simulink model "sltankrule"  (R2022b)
settings: Solver=ode45  StartTime=0  StopTime=Inf  MaxStep=0.2  RelTol=1e-3  AbsTol=1e-6
PreLoadFcn:
  | tank = readfis('tank');
libraries: fuzblock x1, slpidlib x1

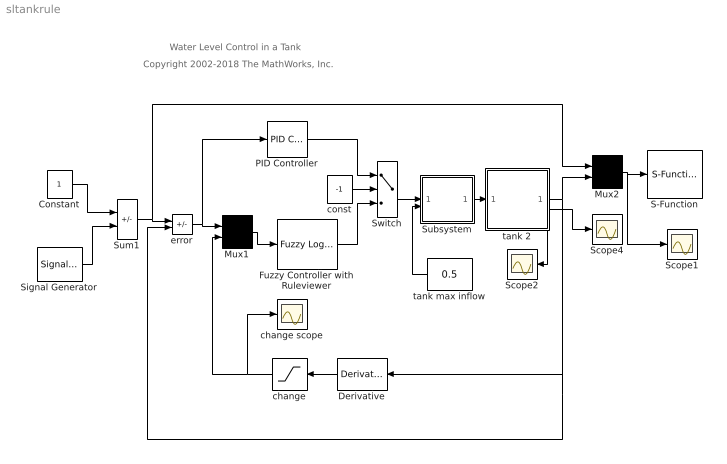
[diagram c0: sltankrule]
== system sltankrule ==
  note: Water Level Control in a Tank
  note: Copyright 2002-2018 The MathWorks, Inc.
  Constant : Constant
  Derivative : Derivative
  Fuzzy Controller with Ruleviewer : fuzblock/Fuzzy Logic  Controller  with Ruleviewer  fismatrix=tank  Ts=2
  Mux1 : Mux  Inputs=2
  Mux2 : Mux  Inputs=2
  PID Controller : slpidlib/PID Controller  Controller=PID  Form=Parallel  TimeDomain=Continuous-time  UseExternalTs=off  SampleTime=1  IntegratorMethod=Forward Euler  FilterMethod=Forward Euler  ControllerParametersSource=internal  P=2  I=0  UseKiTs=off  D=1  N=100  UseFilter=on  TunerSelectOption=Transfer Function Based (PID Tuner App)  InitialConditionSource=internal  InitialConditionForIntegrator=0  InitialConditionForFilter=0  DifferentiatorICPrevScaledInput=0  ExternalReset=none  TrackingMode=off  Kt=1  LimitOutput=off  SatLimitsSource=internal  UpperSaturationLimit=inf  LowerSaturationLimit=-inf  LinearizeAsGain=off  AntiWindupMode=none  Kb=1  LimitIntegrator=off  UpperIntegratorSaturationLimit=inf  LowerIntegratorSaturationLimit=-inf  POutMin=[]  POutMax=[]  IOutMin=[]  IOutMax=[]  DOutMin=[]  DOutMax=[]  NOutMin=[]  NOutMax=[]  SumOutMin=[]  SumOutMax=[]  SaturationOutMin=[]  SaturationOutMax=[]  PParamMin=[]  PParamMax=[]  IParamMin=[]  IParamMax=[]  DParamMin=[]  DParamMax=[]  NParamMin=[]  NParamMax=[]  KbParamMin=[]  KbParamMax=[]  KtParamMin=[]  KtParamMax=[]  KbOutMin=[]  KbOutMax=[]  KtOutMin=[]  KtOutMax=[]  IntegratorOutMin=[]  IntegratorOutMax=[]  FilterOutMin=[]  FilterOutMax=[]  SumI1OutMin=[]  SumI1OutMax=[]  SumI2OutMin=[]  SumI2OutMax=[]  SumI3OutMin=[]  SumI3OutMax=[]  SumI4OutMin=[]  SumI4OutMax=[]  SumDOutMin=[]  SumDOutMax=[]  DifferentiatorOutMin=[]  DifferentiatorOutMax=[]  FilterDiffOutCoefMin=[]  FilterDiffOutCoefMax=[]  ReciprocalOutMin=[]  ReciprocalOutMax=[]  SumDenOutMin=[]  SumDenOutMax=[]  SumNumOutMin=[]  SumNumOutMax=[]  DivideOutMin=[]  DivideOutMax=[]  UdiffTsProdOutMin=[]  UdiffTsProdOutMax=[]  NTsProdOutMin=[]  NTsProdOutMax=[]  UintegralTsProdOutMin=[]  UintegralTsProdOutMax=[]  UngainTsProdOutMin=[]  UngainTsProdOutMax=[]  ClampingZeroOutDataTypeStr=Inherit: Inherit via back propagation  ClampingZeroOutMin=[]  ClampingZeroOutMax=[]  FilterDenConstantOutDataTypeStr=Inherit: Inherit via back propagation  FilterDenConstantOutMin=[]  FilterDenConstantOutMax=[]  PCopyOutDataTypeStr=Inherit: Inherit via back propagation  PCopyOutMin=[]  PCopyOutMax=[]  NCopyOutDataTypeStr=Inherit: Inherit via back propagation  NCopyOutMin=[]  NCopyOutMax=[]  IntegratorContinuousStateAttributes=''  IntegratorStateMustResolveToSignalObject=off  IntegratorRTWStateStorageClass=Auto  FilterContinuousStateAttributes=''  FilterStateMustResolveToSignalObject=off  FilterRTWStateStorageClass=Auto  ParallelPVariant=InternalParameters  IdealPVariant=Disabled  IVariant=InternalParameters  DVariant=InternalParameters  IntegratorVariant=Continuous  SatVariant=Disabled  AWVariant=Passthrough  PCopyVariant=Disabled  TRVariant=Disabled  FdbkBlocksVariant=Forward  IdealPFdbkVariant=Disabled  SatFdbkVariant=Disabled  DerivativeFilterVariant=ContFilter  NVariant=InternalParameters  NCopyVariant=Disabled  FilterICVariant=InternalICsFilter  IntegratorICVariant=InternalICs  ExternalResetVariant=Disabled  TRSumVariant=Passthrough  SumFdbkVariant=Disabled  SumVariant=Sum_PID  TsampFilterVariant=InternalTs  TsampNgainVariant=Passthrough  TsampIntegralVariant=Passthrough  ExternalSaturationOutDataTypeStr=Inherit: Same as second input
  S-Function : S-Function  FunctionName=animtank  Parameters=1  SFunctionDeploymentMode=off  EnableBusSupport=off
  Scope1 : Scope
  Scope2 : Scope
  Scope4 : Scope
  Signal Generator : SignalGenerator  WaveForm=square  Amplitude=0.500000  Frequency=0.100000  Units=rad/sec
  Subsystem : Subsystem  mask(Valve){InitialPosition=0}
      mask prompts: InitialPosition "Initial position [0=closed 1=open]:"
      mask help: Valve
  Sum1 : Sum  Inputs=+-  InputSameDT=on  SaturateOnIntegerOverflow=on
  Switch : Switch
  change : Saturate  UpperLimit=0.1  LowerLimit=-0.1
  change scope : Scope
  const : Constant  Value=-1
  error : Sum  Inputs=+-  InputSameDT=on  SaturateOnIntegerOverflow=on
  tank 2 : Subsystem  mask(Water tank){ht=2, area=1, outletArea=0.05, overflowLimit=0, initialHt=0.5}
      mask prompts: ht "Height of tank (m):"; area "Bottom area (m^2):"; outletArea "Out pipe crossection (m^2):"; overflowLimit "Overflow sensor distance from top (m):"; initialHt "Initial level height (m):"
      mask help: Cylindrical water tank with overflow signal
  tank max inflow : Constant  Value=0.5
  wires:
  tank 2/2(flow out) -> Scope4/1
  tank max inflow/1 -> Subsystem/2(source flow)
  Derivative/1 -> change/1
  Mux1/1 -> Fuzzy Controller with Ruleviewer/1
  change/1 -> Mux1/2, change scope/1
  Constant/1 -> Sum1/1
  Signal Generator/1 -> Sum1/2
  Subsystem/1(out flow) -> tank 2/1(flow in)
  tank 2/1(water level) -> Mux2/2, error/2, Derivative/1
  Sum1/1 -> error/1, Mux2/1
  tank 2/3(overflow flag) -> Scope2/1
  Switch/1 -> Subsystem/1(control)
  Mux2/1 -> S-Function/1, Scope1/1
  error/1 -> Mux1/1, PID Controller/1
  Fuzzy Controller with Ruleviewer/1 -> Switch/3
  PID Controller/1 -> Switch/1
  const/1 -> Switch/2

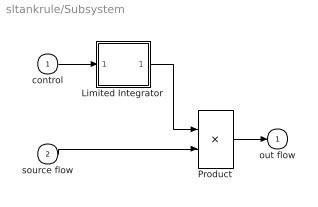
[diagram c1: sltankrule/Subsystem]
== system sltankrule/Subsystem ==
  control : Inport
  source flow : Inport  Port=2
  Limited Integrator : Subsystem  mask(Limited integrator.){lb=0, ub=1, xi=InitialPosition}
      mask prompts: lb "Lower bound:"; ub "Upper bound:"; xi "Initial condition"
      mask help: Limited integrator
  Product : Product  InputSameDT=on  RndMeth=Zero  SaturateOnIntegerOverflow=on
  out flow : Outport  InitialOutput=0  VectorParamsAs1DForOutWhenUnconnected=off
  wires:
  source flow/1 -> Product/2
  Product/1 -> out flow/1
  control/1 -> Limited Integrator/1(In_1)
  Limited Integrator/1(Out_1) -> Product/1

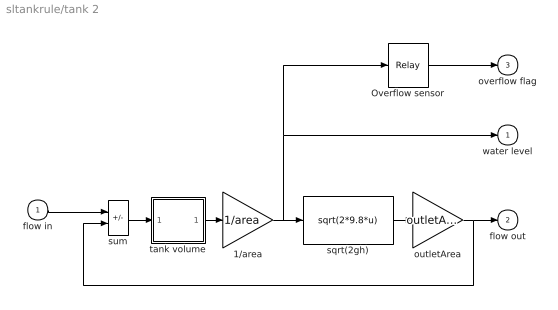
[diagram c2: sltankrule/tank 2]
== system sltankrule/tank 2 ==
  flow in : Inport
  1/area : Gain  Gain=1/area  SaturateOnIntegerOverflow=on
  Overflow sensor : Relay  OnSwitchValue=ht - overflowLimit  OffSwitchValue=ht - overflowLimit
  outletArea : Gain  Gain=outletArea  SaturateOnIntegerOverflow=on
  sqrt(2gh) : Fcn  Expr=sqrt(2*9.8*u)
  sum : Sum  Inputs=+-  InputSameDT=on  SaturateOnIntegerOverflow=on
  tank volume : Subsystem  mask(Limited integrator.){lb=0, ub=ht * area, xi=initialHt * area}
      mask prompts: lb "Lower bound:"; ub "Upper bound:"; xi "Initial condition"
      mask help: Limited integrator
  water level : Outport  InitialOutput=0  VectorParamsAs1DForOutWhenUnconnected=off
  flow out : Outport  Port=2  InitialOutput=0  VectorParamsAs1DForOutWhenUnconnected=off
  overflow flag : Outport  Port=3  InitialOutput=0  VectorParamsAs1DForOutWhenUnconnected=off
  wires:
  outletArea/1 -> flow out/1, sum/2
  sqrt(2gh)/1 -> outletArea/1
  1/area/1 -> Overflow sensor/1, water level/1, sqrt(2gh)/1
  tank volume/1(Out_1) -> 1/area/1
  Overflow sensor/1 -> overflow flag/1
  flow in/1 -> sum/1
  sum/1 -> tank volume/1(In_1)

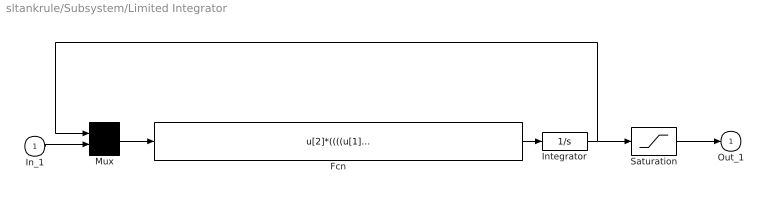
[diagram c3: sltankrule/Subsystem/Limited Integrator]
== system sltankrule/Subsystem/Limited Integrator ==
  In_1 : Inport
  Fcn : Fcn  Expr=u[2]*((((u[1]>lb)+(u[2]>=0))>0) * (((u[1]<ub)+(u[2]<=0))>0))
  Integrator : Integrator  InitialCondition=xi
  Mux : Mux  Inputs=2
  Saturation : Saturate  UpperLimit=ub  LowerLimit=lb
  Out_1 : Outport  InitialOutput=0  VectorParamsAs1DForOutWhenUnconnected=off
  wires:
  Integrator/1 -> Saturation/1, Mux/1
  Fcn/1 -> Integrator/1
  Mux/1 -> Fcn/1
  In_1/1 -> Mux/2
  Saturation/1 -> Out_1/1

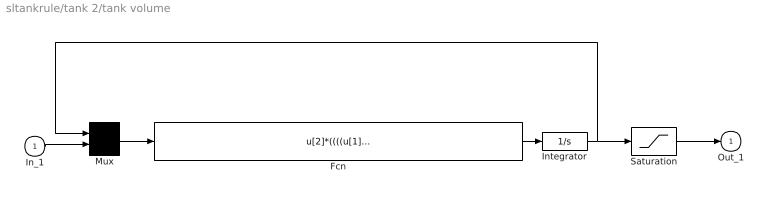
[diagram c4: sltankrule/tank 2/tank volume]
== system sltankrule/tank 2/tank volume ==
  In_1 : Inport
  Fcn : Fcn  Expr=u[2]*((((u[1]>lb)+(u[2]>=0))>0) * (((u[1]<ub)+(u[2]<=0))>0))
  Integrator : Integrator  InitialCondition=xi
  Mux : Mux  Inputs=2
  Saturation : Saturate  UpperLimit=ub  LowerLimit=lb
  Out_1 : Outport  InitialOutput=0  VectorParamsAs1DForOutWhenUnconnected=off
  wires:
  Integrator/1 -> Saturation/1, Mux/1
  Fcn/1 -> Integrator/1
  Mux/1 -> Fcn/1
  In_1/1 -> Mux/2
  Saturation/1 -> Out_1/1
